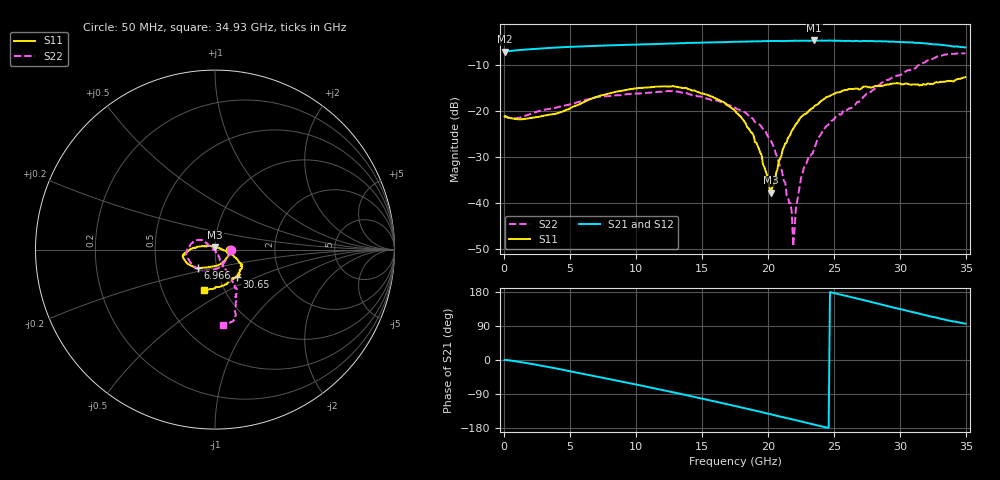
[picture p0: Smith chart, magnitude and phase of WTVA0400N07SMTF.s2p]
! 50 ohm 2-Port S-parameters measured by Modelithics Inc support@modelithics.com  Tampa, FL USA 813-866-6335 (February 2024)
! Smiths Interconnect,  4dB P/N: WTVA0400N07SMTF, Temperature: -50 C
! Board: 10 mil Rogers 4350B, Mounting Pad Dimensions: Length: 15 mils, Width: 25 mils, Gap: 40 mils.
# Hz S RI R 50
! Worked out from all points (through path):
!   352 points, 50 MHz to 34.93 GHz, reference 50 ohm
!   highest |S21| = -4.77 dB at 23.48 GHz (marker M1); lowest = -7.2 dB at 50 MHz (marker M2)
!   group delay of S21, straight-line fit = 21.7 ps
!   lowest |S11| = -37.9 dB at 20.2 GHz (marker M3), VSWR 1.03, Z = 50.1 + j1.28 ohm
!   |S11| at or under -10 dB: start of sweep to end of sweep
!   |S22| runs from -49.5 to -7.5 dB; largest |S21 - S12| = 0.0033
!   S11 on the Smith chart (normalised r, x): 50 MHz: 1.19, -0.01; 6.966 GHz: 0.81, -0.17; 30.65 GHz: 1.21, -0.38; 34.93 GHz: 0.81, -0.38
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5e7  0.0859 -0.00375  0.4358 0.000787  0.4357 0.000518  0.0873 -0.00385
2.4885e9  0.0334 -0.0777  0.4575 -0.104  0.4571 -0.1039  0.0381 -0.0891
5.8715e9  -0.0652 -0.1009  0.4054 -0.2891  0.4051 -0.289  -0.0459 -0.1183
6.966e9  -0.0966 -0.1016  0.3685 -0.3449  0.3682 -0.3447  -0.0727 -0.119
1.1742e10  -0.1757 -0.0484  0.1151 -0.5171  0.1143 -0.517  -0.1534 -0.0455
1.44285e10  -0.1643 -0.0168  -0.0704 -0.5401  -0.0712 -0.5397  -0.1448 0.0139
1.7513e10  -0.0977 0.0161  -0.2935 -0.4763  -0.2937 -0.4758  -0.0925 0.0546
1.8906e10  -0.0469 0.0237  -0.3832 -0.4133  -0.3831 -0.413  -0.0621 0.048
1.9503e10  -0.0246 0.0215  -0.416 -0.3824  -0.4158 -0.3821  -0.0521 0.0402
2.01995e10  0.000981 0.0128  -0.4565 -0.3394  -0.4561 -0.3393  -0.0388 0.0267
2.1095e10  0.0374 0.00382  -0.4958 -0.2777  -0.4957 -0.2772  -0.0181 0.00829
2.1692e10  0.0552 -0.00619  -0.5193 -0.2366  -0.5191 -0.2361  -0.00985 -0.00112
2.17915e10  0.0602 -0.00861  -0.523 -0.2292  -0.5227 -0.2291  -0.00735 -0.00172
2.1891e10  0.0627 -0.00933  -0.5263 -0.2229  -0.5261 -0.2226  -0.00249 -0.00226
2.209e10  0.0701 -0.0108  -0.5346 -0.2066  -0.5345 -0.206  0.00193 -0.00822
2.2488e10  0.083 -0.0181  -0.5452 -0.1765  -0.5451 -0.1756  0.00717 -0.0171
2.33835e10  0.1011 -0.0329  -0.566 -0.1056  -0.5657 -0.1052  0.0169 -0.0301
2.3483e10  0.1048 -0.0349  -0.5693 -0.0961  -0.569 -0.0959  0.0198 -0.0334
2.47765e10  0.1317 -0.0653  -0.5744 0.0173  -0.5741 0.0175  0.0335 -0.0696
2.91545e10  0.1338 -0.1356  -0.4366 0.3496  -0.4359 0.3499  0.1022 -0.1907
3.0647e10  0.1202 -0.1507  -0.3437 0.428  -0.3431 0.4282  0.1157 -0.2487
3.49255e10  -0.0599 -0.2226  -0.0504 0.4832  -0.0483 0.483  0.042 -0.4181
